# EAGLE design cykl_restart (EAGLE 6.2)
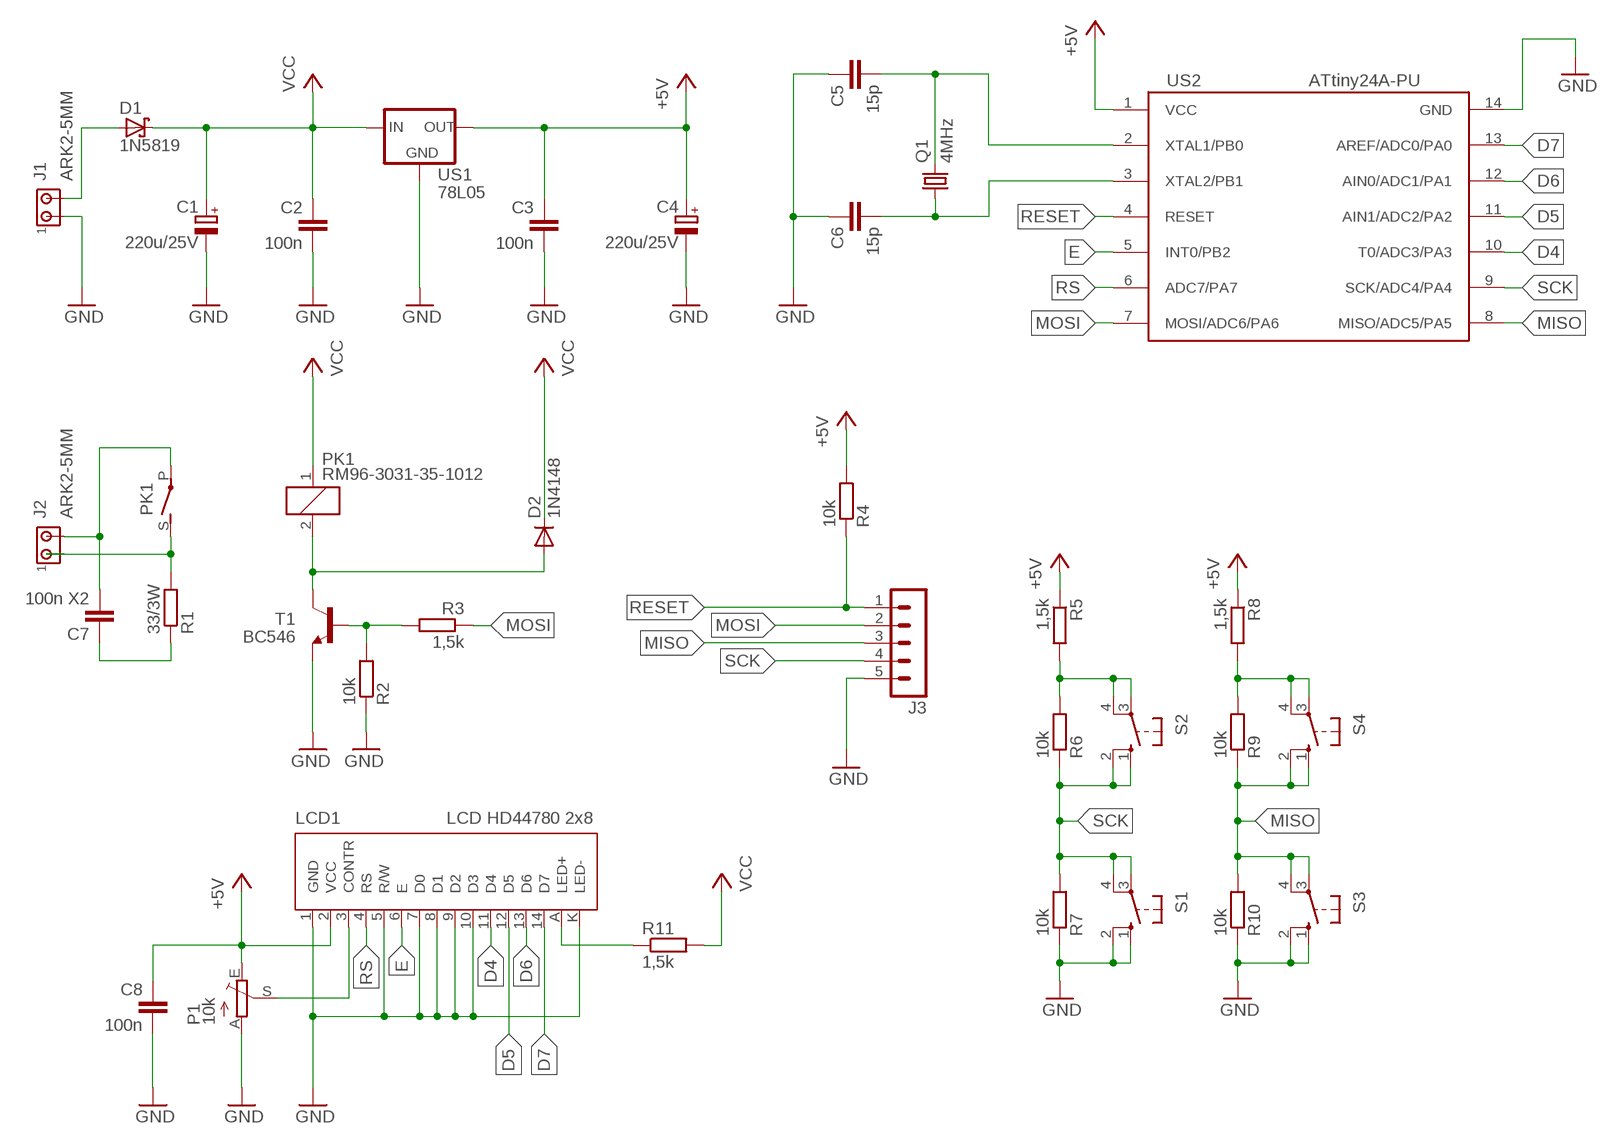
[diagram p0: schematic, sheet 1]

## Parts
C1  220u/25V  CPOL-EUE2.5-7  [E2,5-7]
C2  100n  C-EU050-025X075  [C050-025X075]
C3  100n  C-EU050-025X075  [C050-025X075]
C4  220u/25V  CPOL-EUE2.5-7  [E2,5-7]
C5  15p  C-EU050-025X075  [C050-025X075]
C6  15p  C-EU050-025X075  [C050-025X075]
C7  100n X2  C-EU102_152-062X184  [C102_152-062X184]
C8  100n  C-EU050-025X075  [C050-025X075]
D1  1N5819  SCHOTTKY-DIODEF126Z12  [F126Z12]
D2  1N4148  BAT81  [DO34-7]
J1  ARK2-5MM  [2PIN-5MM]
J2  ARK2-5MM  [2PIN-5MM]
J3  MA05-1  [MA05-1]
LCD1  LCD HD44780 2x8  LCD_ZLACZE-MINI  [LCD_HD44780_1X6_NAD-ELEMENTAMI_Z-PODSW]
P1  10k  TRIM_EU-CA6V  [CA6V]
PK1  RM96-3031-35-1012  RM96  [RM96]
Q1  4MHz  CRYSTALHC49U-V  [HC49U-V]
R1  33/3W  R-EU_0617/17  [0617/17]
R2  10k  R-EU_0207/7  [0207/7]
R3  1,5k  R-EU_0207/7  [0207/7]
R4  10k  R-EU_0207/7  [0207/7]
R5  1,5k  R-EU_0207/7  [0207/7]
R6  10k  R-EU_0207/7  [0207/7]
R7  10k  R-EU_0207/7  [0207/7]
R8  1,5k  R-EU_0207/7  [0207/7]
R9  10k  R-EU_0207/7  [0207/7]
R10  10k  R-EU_0207/7  [0207/7]
R11  1,5k  R-EU_0207/7  [0207/7]
S1  10-XX  [B3F-10XX]
S2  10-XX  [B3F-10XX]
S3  10-XX  [B3F-10XX]
S4  10-XX  [B3F-10XX]
T1  BC546  BC546A  [TO92-EBC]
US1  78L05  78LXX  [78LXX]
US2  ATtiny24A-PU  ATTINY24/44/84-PU  [DIL14]

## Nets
+5V: C3.1 C4.+ C8.1 LCD1.2(VCC) P1.E R4.2 R5.1 R8.1 US1.OUT US2.1(VCC)
D4: LCD1.11(D4) US2.10(T0/ADC3/PA3)
D5: LCD1.12(D5) US2.11(AIN1/ADC2/PA2)
D6: LCD1.13(D6) US2.12(AIN0/ADC1/PA1)
D7: LCD1.14(D7) US2.13(AREF/ADC0/PA0)
E: LCD1.6(E) US2.5(INT0/PB2)
GND: C1.- C2.2 C3.2 C4.- C5.1 C6.1 C8.2 J1.P$1 J3.5 LCD1.1(GND) LCD1.5(R/W) LCD1.7(D0) LCD1.8(D1) LCD1.9(D2) LCD1.10(D3) LCD1.K(LED-) P1.A R2.1 R7.1 R10.1 S1.1(S) S1.2(S1) S3.1(S) S3.2(S1) T1.E US1.GND US2.14(GND)
MISO: J3.3 R9.1 R10.2 S3.3(P) S3.4(P1) S4.1(S) S4.2(S1) US2.8(MISO/ADC5/PA5)
MOSI: J3.2 R3.1 US2.7(MOSI/ADC6/PA6)
N$1: LCD1.3(CONTR) P1.S
N$2: C7.2 J2.P$2 PK1.P(2:P)
N$3: C6.2 Q1.1 US2.3(XTAL2/PB1)
N$4: C5.2 Q1.2 US2.2(XTAL1/PB0)
N$5: R5.2 R6.2 S2.3(P) S2.4(P1)
N$6: LCD1.A(LED+) R11.1
N$7: R2.2 R3.2 T1.B
N$8: D1.A J1.P$2
N$9: D2.A PK1.2 T1.C
N$10: R8.2 R9.2 S4.3(P) S4.4(P1)
N$11: J2.P$1 PK1.S(2:S) R1.2
N$12: C7.1 R1.1
RESET: J3.1 R4.1 US2.4(RESET)
RS: LCD1.4(RS) US2.6(ADC7/PA7)
SCK: J3.4 R6.1 R7.2 S1.3(P) S1.4(P1) S2.1(S) S2.2(S1) US2.9(SCK/ADC4/PA4)
VCC: C1.+ C2.1 D1.C D2.C PK1.1 R11.2 US1.IN

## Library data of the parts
C1 C4 = rcl:CPOL-EU: POLARIZED CAPACITOR, European symbol
C2 C3 C5-C8 = rcl:C-EU: CAPACITOR, European symbol
D1 = diode:SCHOTTKY-DIODE: Schottky Diode
D2 = diode:BAT81: DIODE
J1 J2 = zlacza_futrzak:ARK2: ARK 2
J3 = zlacza_futrzak:MA05-1: PIN HEADER; OC_FARNELL: unknown; OC_NEWARK: unknown
LCD1 = inne_futrzak:LCD_ZLACZE
P1 = pot:TRIM_EU-: POTENTIOMETER
PK1 = inne_futrzak:RM96: RELAY 1 x norm. open, Omron; OC_FARNELL: unknown; OC_NEWARK: unknown
Q1 = crystal:CRYSTAL: CRYSTAL; OC_FARNELL: 1666969; OC_NEWARK: unknown
R1-R11 = rcl:R-EU_: RESISTOR, European symbol
S1-S4 = switch-omron:10-XX: OMRON SWITCH; MPN: B3F-1000; OC_FARNELL: 176432; OC_NEWARK: 36M3542
T1 = transistor-npn:BC546*: NPN Transistor
US1 = v-reg:78LXX: VOLTAGE REGULATOR
US2 = scalaki_futrzak:ATTINY24/44/84

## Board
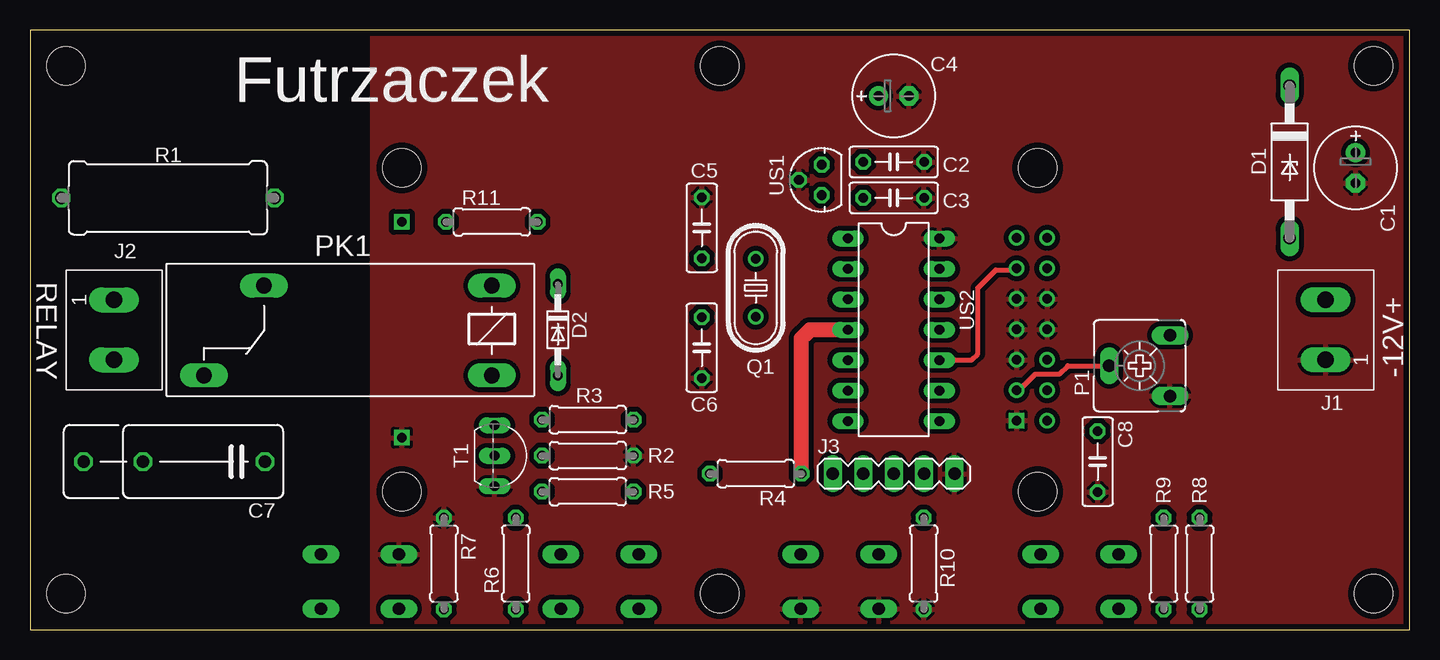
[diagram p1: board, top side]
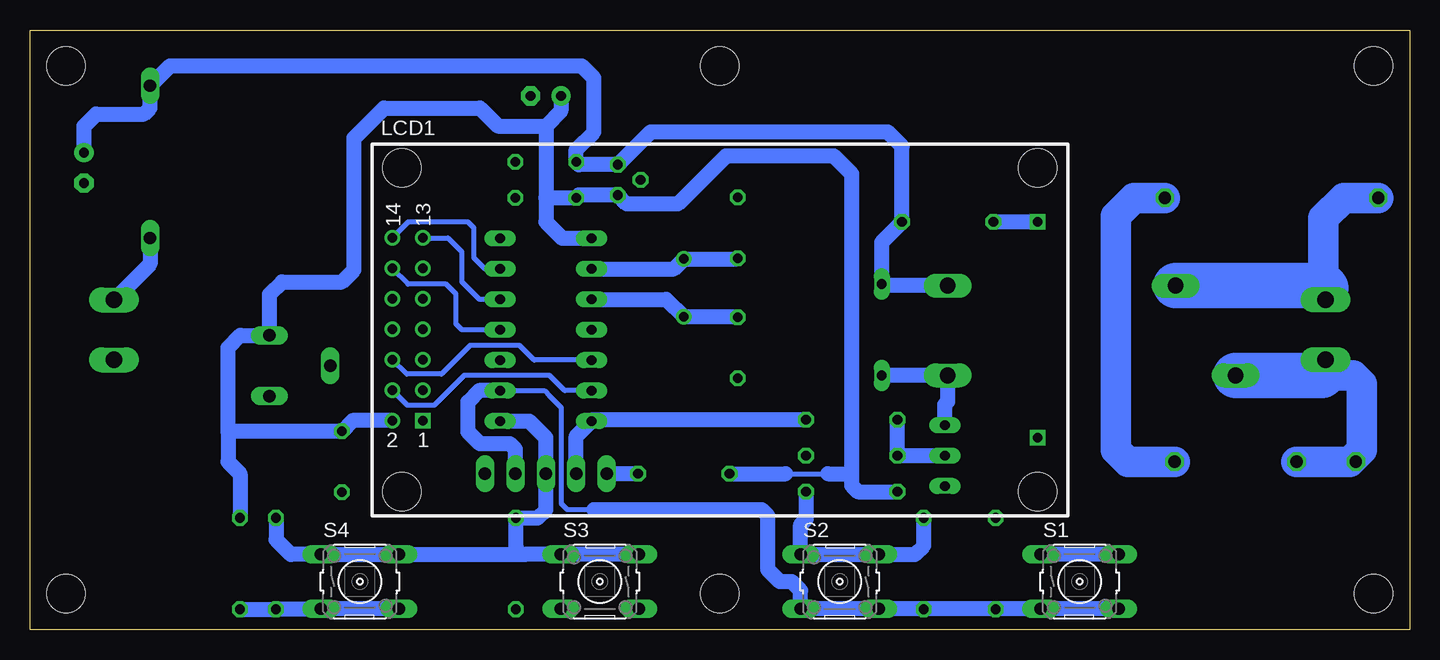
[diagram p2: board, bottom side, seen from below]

Size 115 x 50 mm. Coordinates in mm from the lower left corner, seen from the top.
Outline: 0,0 115,0 115,50 0,50 0,0
Copper layers (1*16): Top 0.035mm / dielectric 1.5mm / Bottom 0.035mm
Design rules: minimum track width 10mil, minimum drill 23mil, track to track 8mil, track to pad 8mil, pad to pad 8mil, via to via 8mil, smd to smd 8mil, copper to edge 20mil, drill to drill 8mil, minimum pad ring 10mil, minimum via ring 8mil, stop-mask expansion 4mil, vias tented up to drill 0mil, thermal gap 10mil
Holes 3.2 mm at 3,3 3,47 112,3 112,47 57.5,3 57.5,47

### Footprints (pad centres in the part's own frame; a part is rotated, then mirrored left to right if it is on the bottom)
E2,5-7 = drill 0.813 pad 1.6: + -1.27,0 | drill 0.813 pad 1.6 octagon: - 1.27,0
C050-025X075 = drill 0.813 octagon: 1 -2.54,0; 2 2.54,0
C102_152-062X184 = drill 1.016 octagon: 1 -5.08,0; 2 5.08,0; 3 10.033,0
F126Z12 = drill 1.016 long: A 6.35,0; C -6.35,0
DO34-7 = drill 0.813 long: A 3.81,0; C -3.81,0
2PIN-5MM = drill 1.4 long: P$1 -2.5,0; P$2 2.5,0
MA05-1 = drill 1.016 long: 1 -5.08,0; 2 -2.54,0; 3 0,0; 4 2.54,0; 5 5.08,0
LCD_HD44780_1X6_NAD-ELEMENTAMI_Z-PODSW = drill 0.8 square: 1 1.74,5.92; A 53,22.5; K 53,4.5 | drill 0.8: 2 -0.8,5.92; 3 1.74,8.46; 4 -0.8,8.46; 5 1.74,11; 6 -0.8,11; 7 1.74,13.54; 8 -0.8,13.54; 9 1.74,16.08; 10 -0.8,16.08; 11 1.74,18.62; 12 -0.8,18.62; 13 1.74,21.16; 14 -0.8,21.16 | hole 3.2: 0,0; 0,27; 53,0; 53,27
CA6V = drill 1.016 long: A -2.54,-2.54; E 2.54,-2.54; S 0,2.54
RM96 = drill 1.321 long: 1 3.5,1.817; 2 3.5,9.31; P 27.5,9.31; S 22.5,1.817
HC49U-V = drill 0.813: 1 -2.413,0; 2 2.413,0
0617/17 = drill 1.016 octagon: 1 -8.89,0; 2 8.89,0
0207/7 = drill 0.813 octagon: 1 -3.81,0; 2 3.81,0
B3F-10XX = drill 1.016 long: 1 -3.251,2.261; 2 3.251,2.261; 3 -3.251,-2.261; 4 3.251,-2.261
TO92-EBC = drill 0.813 long: B 0,-1.27; C -2.54,-1.27; E 2.54,-1.27
78LXX = drill 0.813 octagon: GND 0,1.905; IN 1.27,0; OUT -1.27,0
DIL14 = drill 0.813 long: 1 -7.62,-3.81; 2 -5.08,-3.81; 3 -2.54,-3.81; 4 0,-3.81; 5 2.54,-3.81; 6 5.08,-3.81; 7 7.62,-3.81; 8 7.62,3.81; 9 5.08,3.81; 10 2.54,3.81; 11 0,3.81; 12 -2.54,3.81; 13 -5.08,3.81; 14 -7.62,3.81

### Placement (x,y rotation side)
C1  110.5,38.5 270 top
C2  72,39 0 top
C3  72,36 0 top
C4  72,44.5 0 top
C5  56,33.5 270 top
C6  56,23.5 90 top
C7  14.5,14 180 top
C8  89,14 270 top
D1  105,39 270 top
D2  44,25 270 top
J1  108,25 90 top
J2  7,25 270 top
J3  72,13 0 top
LCD1  84,11.5 0 bottom
P1  92.5,22 90 top
PK1  42,30.5 180 top
Q1  60.5,28.5 90 top
R1  11.5,36 180 top
R2  46.5,14.5 180 top
R3  46.5,17.5 180 top
R4  60.5,13 180 top
R5  46.5,11.5 0 top
R6  40.5,5.5 90 top
R7  34.5,5.5 270 top
R8  97.5,5.5 270 top
R9  94.5,5.5 270 top
R10  74.5,5.5 90 top
R11  38.5,34 0 top
S1  27.5,4 0 bottom
S2  47.5,4 180 bottom
S3  67.5,4 180 bottom
S4  87.5,4 0 bottom
T1  40,14.5 270 top
US1  66,37.5 90 top
US2  72,25 270 top

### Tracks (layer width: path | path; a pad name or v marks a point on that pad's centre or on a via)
+5V
  Bottom 0.406: 52,13 48.5,13
  Bottom 1.27: C4.+ 70.73,43.27 72,42 | 72,42 72,36 | 72,36 72,34 70.62,32.62 US2.1 | 72,36 C3.1 69.23,36.23 US1.OUT 65.27,35.5 61,35.5 57,39.5 48,39.5 46.5,38 46.5,13 | 72,42 76,42 77.5,43.5 85.5,43.5 88,41 88,30 89,29 94,29 95.04,27.96 P1.E 97.46,24.54 98.5,23.5 98.5,16.5 | LCD1.2 88.12,17.42 C8.1 98.46,16.54 98.5,16.5 | 98.5,16.5 98.5,14 97.5,13 R8.1 | R5.1 46,11.5 46.5,12 46.5,13 | R4.2 52,13 | 48.5,13 46.5,13
D4
  Top 0.406: US2.10 78.46,22.46 79,23 79,28.5 80.5,30 82.14,30 LCD1.11
D5
  Bottom 0.406: US2.11 79,25 79.5,25.5 79.5,28 80.3,28.8 83.48,28.8 LCD1.12
D6
  Bottom 0.406: US2.12 77.54,27.54 78,28 79,29 79,31.5 80,32.5 80.16,32.66 LCD1.13
D7
  Bottom 0.406: US2.13 77.08,30.08 78,31 78,33.5 78.5,34 83.46,34 LCD1.14
E
  Bottom 0.406: US2.5 72.96,22.46 74.2,23.7 78.3,23.7 80.7,21.3 83.6,21.3 LCD1.6
GND
  Bottom 1.27: S1.2 S1.1
  pour Top (isolate 0.406): 28.5,0 115,0 115,50 28.5,50
MISO
  Bottom 1.27: S3.3 S3.4 73.76,6.26 74.5,6.26 | 74.5,6.26 S4.2 S4.1 93.26,6.26 93.5,6.5 94.5,7.5 R9.1 | 74.5,6.26 74.5,7 R10.2 72.69,9.31 72,10 J3.3 72,16 73,17 73.38,17.38 US2.8
MOSI
  Bottom 1.27: R3.1 68.07,17.5 US2.7 69.46,16.11 J3.2
N$1
  Top 0.406: LCD1.3 82.46,19.96 83.8,21.3 85.8,21.3 86.5,22 P1.S
N$2
  Bottom 1.27: 7,21.5 J2.P$2
  Bottom 2.54: 7.31,21.19 4.69,21.19 4,20.5 4,15 5,14 C7.2
  Bottom 3.81: PK1.P 7.31,21.19 7,21.5
N$3
  Bottom 1.27: US2.3 61.95,27.54 Q1.1 56.05,26.09 C6.2
N$4
  Bottom 1.27: US2.2 61.33,30.08 Q1.2 56.05,30.91 C5.2
N$5
  Bottom 1.27: R6.2 40.5,7 41.24,6.26 S2.3 S2.4 50.75,8.75 50.31,9.19 R5.2
N$6
  Bottom 1.27: LCD1.A R11.1
N$7
  Bottom 1.27: T1.B R2.2 R3.2
N$8
  Bottom 1.27: D1.A 105,30.5 J1.P$2
N$9
  Bottom 1.27: D2.A PK1.2 38.5,19 38.73,18.77 T1.C
N$10
  Bottom 1.27: S4.4 S4.3 90.8,1.69 R9.2 R8.2
N$11
  Bottom 1.27: 7,28.5 J2.P$1
  Bottom 2.54: 7.18,28.68 7.18,34.32 5.5,36 R1.2
  Bottom 3.81: PK1.S 7.18,28.68 7,28.5
N$12
  Bottom 2.54: R1.1 23,36 24.5,34.5 24.5,15 23.5,14 C7.1
RESET
  Top 1.27: US2.4 65,25 64.5,24.5 64.31,24.31 R4.1
  Bottom 1.27: R4.1 J3.1
RS
  Bottom 0.406: US2.6 70.42,19.92 71.7,21.2 78.8,21.2 81.3,18.7 83.54,18.7 LCD1.4
SCK
  Bottom 0.406: 68,10 70.2,10 70.7,10.5 70.7,18.5 71.7,19.5 72.12,19.92 US2.9
  Bottom 1.27: S1.4 S1.3 34.5,1.74 | 34.5,1.74 40.5,1.74 | 40.5,1.74 S2.1 S2.2 50.75,3.25 51.5,4 52.5,4 53.5,5 53.5,9.5 54,10 68,10 | R7.2 34.5,1.74 | R6.1 40.5,1.74 | J3.4 74.54,15.04 75,15.5 77.5,15.5 78.5,16.5 78.5,19 77.58,19.92 US2.9
VCC
  Bottom 1.27: C1.+ 110.5,42 109.5,43 105.5,43 105,43.5 D1.C 103.35,47 69,47 68,46 68,41.5 69.46,40.04 C2.1 69.23,38.77 US1.IN 63.27,41.5 43.5,41.5 42.31,40.31 R11.2 44,32.31 D2.C 43.87,28.68 PK1.1

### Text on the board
tPlace: Futrzaczek | RELAY | -12V+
